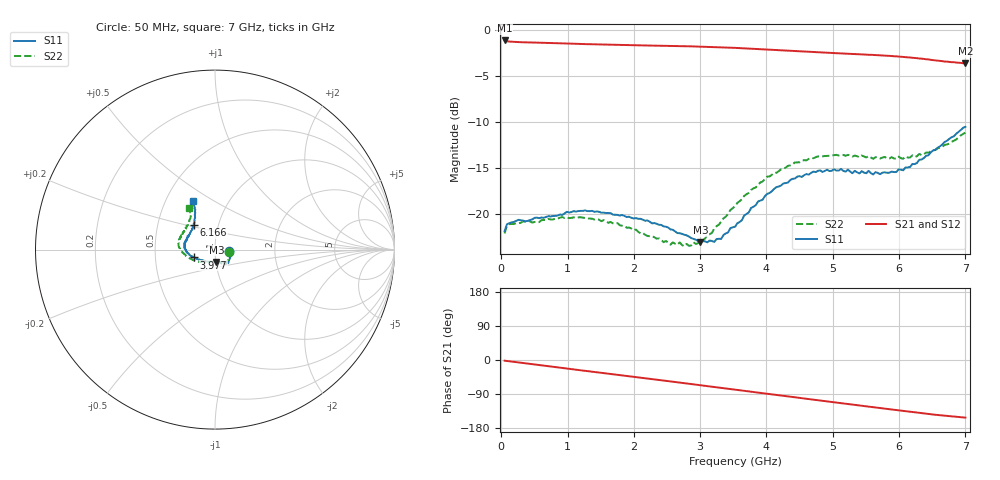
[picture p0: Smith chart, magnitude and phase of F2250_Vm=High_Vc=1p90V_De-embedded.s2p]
! Integrated Device Technology
! Corporate Headquarters
! 6024 Silver Creek Valley Road
! San Jose, CA 95138  USA
! Phone:  1-408-284-8200
! Toll Free:  1-800-223-1366
! Webpage:  http://www.idt.com/
! Timing and RF Division
! 515 Groton Road, Suite 102
! Westford, MA 01886-6024
! Device:  F2250
! Description: Voltage Variable RF Attenuator
! Frequency:  50.0 -  6000.00 MHz
! Package:  3x3 mm Thin QFN Plastic Package: 16 pin
! Ports:  2 RF, 3 DC
!  Pin  1  = GND
!  Pin  2  = NC
!  Pin  3  = RF1  = Port 1
!  Pin  4  = NC
!  Pin  5  = GND
!  Pin  6  = GND
!  Pin  7  = GND
!  Pin  8  = GND
!  Pin  9  = NC
!  Pin 10  = RF2  = Port 2
!  Pin 11  = NC
!  Pin 12  = GND
!  Pin 13  = GND
!  Pin 14  = VCNTRL
!  Pin 15  = VDD
!  Pin 16  = VMODE
! Vcntrl:  1.900 Volts
! Vmode:  +3.300 Volts
! Vdd:  +3.30  Volts
! Current:  1.323 mA
! Data:  The device was measured on a the F2250 evaluation board which has
!  individual transmission lines to the RF pins.  Data was collected
!  using a calibrated network analyzer.  The evaluation board was
!  de-embedded using a TRL calibration technique.
!  The reference plane is the edge of the package pin.
! Misc:  SN 10
!  Action Tracker AT0258
! Date Measured:  2014-11-26
! Date:  2015-10-15  MJV
! Note:
!  Integrated Device Technology supplies this data as a sample of measured
!  data at the package pin for this product.  Your particular data for this
!  product may vary.
!  Data was taken at 25 degrees C.
!  Integrated Device Technology reserves the right to change this data at anytime.
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# GHz S dB R 50
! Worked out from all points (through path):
!   201 points, 50 MHz to 7 GHz, reference 50 ohm
!   highest |S21| = -1.17 dB at 50 MHz (marker M1); lowest = -3.6 dB at 7 GHz (marker M2)
!   group delay of S21, straight-line fit = 61.1 ps
!   lowest |S11| = -23.1 dB at 3.004 GHz (marker M3), VSWR 1.15, Z = 50.2 - j7 ohm
!   |S11| at or under -10 dB: start of sweep to end of sweep
!   |S22| runs from -23.5 to -11.2 dB; largest |S21 - S12| = 0.0018
!   S11 on the Smith chart (normalised r, x): 50 MHz: 1.17, -0.02; 3.977 GHz: 0.79, -0.07; 6.166 GHz: 0.76, +0.21; 7 GHz: 0.68, +0.40
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0.05  -21.91 -7.0  -1.17 -1.8  -1.16 -1.8  -22.15 -8.0
0.08475  -21.17 -6.6  -1.25 -2.5  -1.25 -2.5  -21.33 -7.3
0.1195  -21.04 -7.3  -1.29 -3.3  -1.28 -3.3  -21.16 -7.2
0.328  -20.75 -14.6  -1.36 -7.9  -1.36 -7.9  -20.85 -15.8
1.2315  -19.70 -46.8  -1.56 -27.9  -1.55 -27.9  -20.44 -54.5
1.75275  -20.14 -53.8  -1.65 -39.1  -1.65 -39.1  -21.03 -63.8
2.37825  -21.22 -55.8  -1.74 -52.7  -1.74 -52.7  -22.70 -71.1
2.552  -21.72 -59.5  -1.75 -56.5  -1.75 -56.5  -23.38 -77.6
2.7605  -22.30 -66.6  -1.79 -61.2  -1.79 -61.2  -23.54 -87.8
3.00375  -23.13 -84.0  -1.83 -66.6  -1.83 -66.7  -22.86 -106.7
3.1775  -22.98 -97.3  -1.87 -70.6  -1.87 -70.6  -22.09 -120.1
3.3165  -22.76 -113.8  -1.91 -73.7  -1.91 -73.8  -20.87 -130.3
3.4555  -21.57 -127.4  -1.95 -76.9  -1.95 -76.9  -19.60 -138.8
3.525  -21.44 -132.2  -1.97 -78.4  -1.97 -78.5  -19.19 -142.3
3.97675  -18.10 -159.5  -2.14 -88.6  -2.15 -88.7  -16.24 -163.1
4.4285  -16.18 -173.9  -2.32 -98.6  -2.33 -98.6  -14.44 -177.6
4.7065  -15.43 178.2  -2.42 -104.7  -2.42 -104.7  -13.98 176.2
5.054  -15.32 169.8  -2.55 -112.4  -2.55 -112.4  -13.61 168.6
5.85325  -15.55 142.9  -2.85 -129.9  -2.85 -130.0  -14.01 149.2
6.166  -14.92 131.0  -3.02 -136.7  -3.02 -136.8  -13.89 140.6
6.54825  -13.04 120.5  -3.32 -144.6  -3.33 -144.7  -13.08 128.4
7  -10.56 114.7  -3.65 -152.0  -3.66 -152.1  -11.20 121.8
